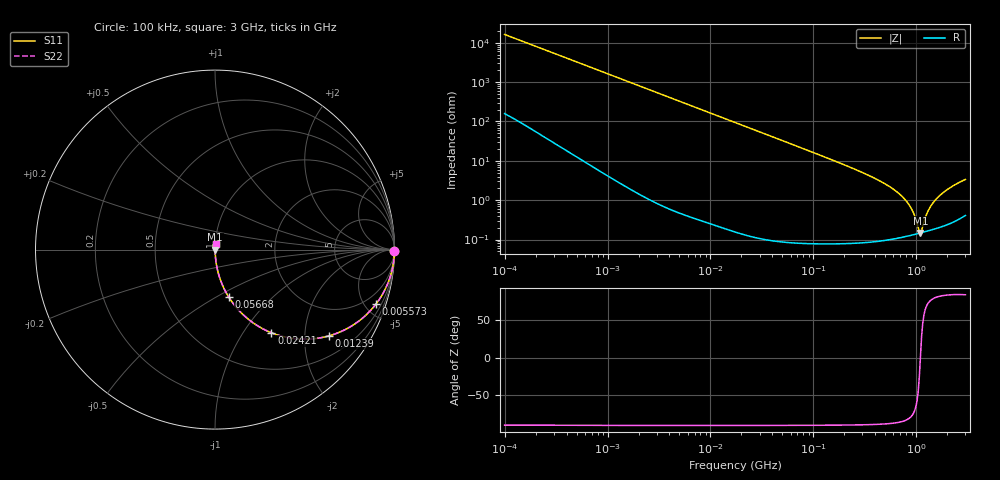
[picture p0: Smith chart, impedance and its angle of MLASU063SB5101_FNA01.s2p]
! MLASU063SB5101_FNA01  S-PARAMETER MODEL  ( Standard Model )
! Model Generated by TAIYO YUDEN Corporation (http://www.ty-top.com)
! Version 1.0
! TAIYO YUDEN Control No. 220601
! Copyright(c) 2012 TAIYO YUDEN CO.,LTD. All Rights Reserved.
! Product Description (link to TY-COMPAS)
! https://ds.yuden.co.jp/TYCOMPAS/or/detail?pn=MLASU063SB5101KFNA01&u=M
! Products Name : Multilayer Ceramic Capacitors
! Characteristics :
!  Capacitance : 100 [pF] , Rated Voltage : 50 [V] , TCC : B / X5R
!  Case Size : 0.6 x 0.3 / 0.024 x 0.012 [mm/inch] , Thickness : 0.3 / 0.012 [mm/inch]
!  (Conditions: Temperature = 25 [degC] , DC Bias Voltage = 0 [V])
! External Node Assignments :
!  1  o---| |---o  2
! GND o---------o GND
! Frequency Range : 100kHz  -  3GHz  [ 401 STEP ]
# MHZ S RI R 50
! Freq[MHz].  S11 Real  S11 Imag  S21 Real  S21 Imag  S12 Real  S12 Imag  S22 Real  S22 Imag
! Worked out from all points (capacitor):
!   401 points, 100 kHz to 3 GHz, reference 50 ohm
!   read as one part in series: C = 97.9 pF near 105.3 kHz
!   lowest |Z| = 148 mohm at 1.098 GHz (marker M1)
!   series resonance near 1.096 GHz, so ESL is about 220 pH
!   S11 on the Smith chart (normalised r, x): 100 kHz: open; 5.573 MHz: 1.01, -5.87; 12.39 MHz: 1.00, -2.64; 24.21 MHz: 1.00, -1.35; 56.68 MHz: 1.00, -0.58; 3 GHz: 1.01, +0.07
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0.1  0.9999 -0.00616  9.81e-05 0.00616  9.81e-05 0.00616  0.9999 -0.00616
0.562235  0.9987 -0.0344  0.00131 0.0344  0.00131 0.0344  0.9987 -0.0344
3.161081  0.9637 -0.1862  0.0363 0.1862  0.0363 0.1862  0.9637 -0.1862
5.572849  0.8957 -0.3049  0.1043 0.3049  0.1043 0.3049  0.8957 -0.3049
12.38951  0.6357 -0.4805  0.3643 0.4805  0.3643 0.4805  0.6357 -0.4805
17.7727  0.4592 -0.4975  0.5408 0.4975  0.5408 0.4975  0.4592 -0.4975
24.21403  0.3141 -0.4632  0.6859 0.4632  0.6859 0.4632  0.3141 -0.4632
36.57227  0.1673 -0.3722  0.8327 0.3722  0.8327 0.3722  0.1673 -0.3722
56.67997  0.0774 -0.2657  0.9226 0.2657  0.9226 0.2657  0.0774 -0.2657
97.38194  0.0278 -0.1621  0.9722 0.1621  0.9722 0.1621  0.0278 -0.1621
294.964  0.00345 -0.0512  0.9965 0.0512  0.9965 0.0512  0.00345 -0.0512
547.5153  0.00149 -0.0222  0.9985 0.0222  0.9985 0.0222  0.00149 -0.0222
690.4488  0.00131 -0.0141  0.9987 0.0141  0.9987 0.0141  0.00131 -0.0141
826.9535  0.0013 -0.0084  0.9987 0.0084  0.9987 0.0084  0.0013 -0.0084
940.6869  0.00135 -0.0045  0.9986 0.0045  0.9986 0.0045  0.00135 -0.0045
1042.837  0.00142 -0.00145  0.9986 0.00145  0.9986 0.00145  0.00142 -0.00145
1097.999  0.00147 5.73e-05  0.9985 -5.73e-05  0.9985 -5.73e-05  0.00147 5.73e-05
1156.079  0.00153 0.00156  0.9985 -0.00156  0.9985 -0.00156  0.00153 0.00156
1315.078  0.0017 0.00534  0.9983 -0.00534  0.9983 -0.00534  0.0017 0.00534
1575.075  0.00204 0.0108  0.998 -0.0108  0.998 -0.0108  0.00204 0.0108
2091.327  0.00289 0.0199  0.9971 -0.0199  0.9971 -0.0199  0.00289 0.0199
3000  0.00517 0.0331  0.9948 -0.0331  0.9948 -0.0331  0.00517 0.0331
